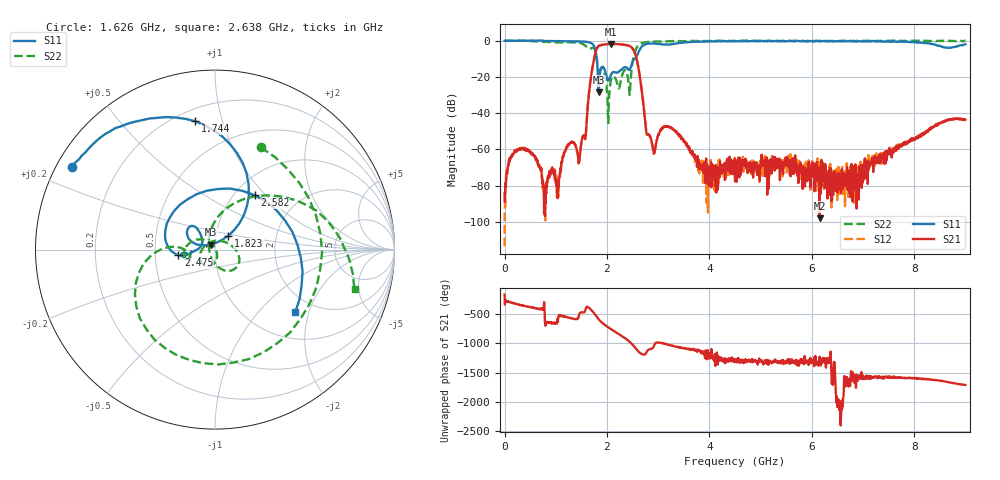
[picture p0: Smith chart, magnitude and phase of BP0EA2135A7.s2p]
!Agilent Technologies,E8358A,US40260310,A.06.04.32
!Agilent E8358A: A.06.04.32
!Date: Friday, May 08, 2020 03:15:27
!Correction: S11(Full 2 Port(1,2)) S21(Full 2 Port(1,2)) S12(Full 2 Port(1,2)) S22(Full 2 Port(1,2))
!S2P File: Measurements: S11, S21, S12, S22:
# Hz S  dB  R 50
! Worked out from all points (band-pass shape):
!   1601 points, 300 kHz to 9 GHz, reference 50 ohm
!   highest |S21| = -1.77 dB at 2.076 GHz (marker M1); lowest = -97.9 dB at 6.154 GHz (marker M2)
!   |S21| within 3 dB of the highest: 1.795 GHz to 2.511 GHz (716.3 MHz wide, 33.3 % of centre)
!   lowest |S11| = -28.6 dB at 1.84 GHz (marker M3), VSWR 1.08, Z = 47.5 + j2.65 ohm
!   |S11| at or under -10 dB: 1.799 GHz to 2.541 GHz (741.8 MHz wide, 34.2 % of centre)
!   |S22| runs from -45.5 to 0.1 dB; largest |S21 - S12| = 0.012
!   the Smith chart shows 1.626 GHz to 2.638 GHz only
!   S11 on the Smith chart (normalised r, x): 1.626 GHz: 0.04, +0.27; 1.744 GHz: 0.27, +0.82; 1.823 GHz: 1.15, +0.18; 2.475 GHz: 0.66, -0.04; 2.582 GHz: 1.23, +0.87; 2.638 GHz: 1.61, -1.63
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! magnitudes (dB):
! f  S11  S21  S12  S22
! 300 kHz  0.0  -84.3  -113.4  0.0
! 242.2 MHz  0.0  -60.4  -60.4  0.0
! 787.8 MHz  -0.1  -96.7  -81.1  -0.6
! 1.502 GHz  -0.4  -55.6  -55.5  -1.5
! 1.626 GHz  -0.7  -35.5  -35.5  -4.1
! 1.744 GHz  -2.8  -10.5  -10.6  -4.2
! 1.823 GHz  -19.4  -3.3  -3.3  -14.4
! 1.84 GHz  -28.6  -2.9  -2.9  -16.7
! 2.076 GHz  -18.9  -1.8  -1.8  -21.9
! 2.475 GHz  -13.7  -3.5  -3.5  -17.3
! 2.582 GHz  -8.5  -10.3  -10.3  -3.8
! 2.638 GHz  -4.9  -19.2  -19.1  -1.8
! 2.79 GHz  -1.7  -52.0  -51.7  -0.8
! 3.004 GHz  -1.8  -52.1  -52.3  -0.4
! 3.28 GHz  -1.8  -48.7  -48.8  -0.2
! 4.112 GHz  -0.3  -79.5  -76.1  -0.1
! 4.5 GHz  -0.2  -77.7  -67.2  -0.2
! 6.002 GHz  -0.2  -73.7  -69.9  -0.2
! 6.154 GHz  -0.2  -97.9  -65.7  0.0
! 6.834 GHz  -0.4  -82.0  -71.7  -0.2
! 7.504 GHz  -0.5  -62.8  -61.1  -0.2
! 9 GHz  -1.9  -43.6  -44.0  -0.1
